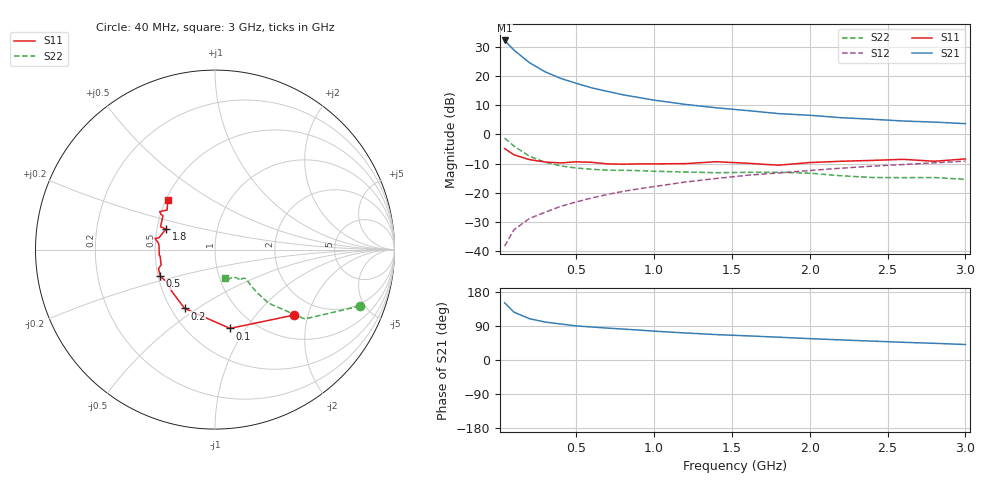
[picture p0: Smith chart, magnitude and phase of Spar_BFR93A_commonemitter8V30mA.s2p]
! Filename:  BFR93AH.S2P  Version:  2.0
! NXP part #: BFR93A  Date: May 1990
! Bias condition: Vce=8V, Ic=30mA
#  MHz  S  MA  R  50
! Freq  S11  S21  S12  S22  !GUM [dB]
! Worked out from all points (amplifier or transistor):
!   21 points, 40 MHz to 3 GHz, reference 50 ohm
!   highest |S21| = 32.3 dB at 40 MHz (marker M1)
!   |S21| within 3 dB of that: start of sweep to 94.22 MHz
!   unconditionally stable (mu >= 1): 660.8 MHz to 2.944 GHz
!   at 300 MHz: K = 0.88, MSG = 24.2 dB, |S12| = -26.7 dB
!   at 1 GHz: K = 1.04, MAG = 13.6 dB, |S12| = -17.9 dB
!   at 3 GHz: K = 0.99, MSG = 6.4 dB, |S12| = -9.2 dB
!   S11 on the Smith chart (normalised r, x): 40 MHz: 1.51, -1.64; 100 MHz: 0.78, -0.85; 200 MHz: 0.59, -0.44; 500 MHz: 0.51, -0.17; 1.8 GHz: 0.56, +0.14; 3 GHz: 0.51, +0.33
40  0.572 -39.6  41.36 151.0  0.012 73.0  0.866 -21.3
100  0.447 -79.2  28.22 126.2  0.023 63.2  0.632 -37.7
200  0.369 -117.3  17.12 109.0  0.036 64.3  0.422 -45.0
300  0.336 -134.9  11.97 100.1  0.046 65.9  0.333 -45.6
400  0.324 -146.6  9.213 95.0  0.058 68.7  0.288 -45.2
500  0.339 -154.1  7.585 90.0  0.069 70.1  0.265 -44.3
600  0.332 -161.4  6.325 87.1  0.081 70.4  0.252 -44.0
700  0.312 -164.2  5.508 84.2  0.093 72.1  0.244 -43.8
800  0.308 -172.9  4.816 81.6  0.105 71.4  0.242 -43.5
900  0.312 -174.5  4.331 79.1  0.116 72.3  0.239 -43.9
1000  0.312 177.6  3.892 76.1  0.127 72.1  0.233 -43.6
1200  0.315 174.0  3.293 71.4  0.152 71.6  0.226 -44.7
1400  0.34 169.3  2.873 67.0  0.175 70.0  0.22 -47.4
1600  0.32 168.3  2.574 63.7  0.199 69.6  0.223 -49.2
1800  0.296 157.3  2.285 60.2  0.218 68.2  0.224 -50.2
2000  0.329 157.2  2.136 56.3  0.24 66.8  0.216 -50.6
2200  0.346 146.9  1.944 53.0  0.263 66.4  0.195 -52.9
2400  0.358 146.9  1.827 49.9  0.285 64.5  0.182 -59.9
2600  0.374 145.5  1.705 46.7  0.304 63.0  0.181 -66.2
2800  0.346 140.4  1.631 44.0  0.326 61.8  0.182 -69.4
3000  0.38 133.9  1.535 40.9  0.348 60.1  0.169 -70.8
